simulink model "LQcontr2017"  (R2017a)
settings: Solver=VariableStepAuto  StartTime=0.0  StopTime=10.0  RelTol=1e-3
InitFcn:
  | initParams
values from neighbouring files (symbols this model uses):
  c = 8e-3    (= 0.008)    [initParams.m]
  g = 9.81    [initParams.m]
  L1 = 0.5    [initParams.m]
  m = 0.2    [initParams.m]
  R = 10    [initParams.m]
  ue = R*xe(3)    [initParams.m]
  x0 = [0.1;0;0.3]    [initParams.m]
  xe = [x1d;0;x1d*sqrt(g*m/c)]    [initParams.m]
undefined symbols (not defined in the file or in its folder): KLQ

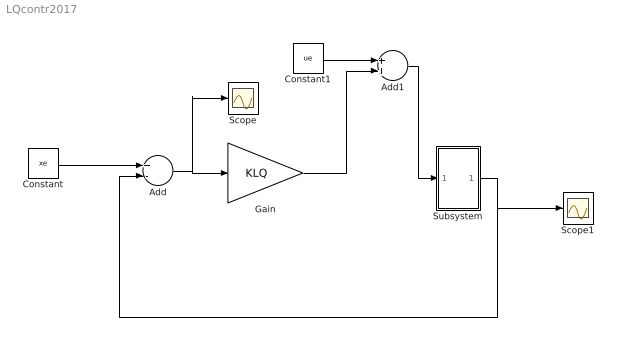
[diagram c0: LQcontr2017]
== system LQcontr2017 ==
  Add : Sum  Inputs=+-
  Add1 : Sum
  Constant : Constant  Value=xe
  Constant1 : Constant  Value=ue
  Gain : Gain  Gain=KLQ  Multiplication=Matrix(K*u) (u vector)
  Scope : Scope
  Scope1 : Scope
  Subsystem : Subsystem
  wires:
  Constant/1 -> Add/1
  Subsystem/1(x) -> Add/2, Scope1/1
  Add/1 -> Scope/1, Gain/1
  Constant1/1 -> Add1/1
  Gain/1 -> Add1/2
  Add1/1 -> Subsystem/1(u)

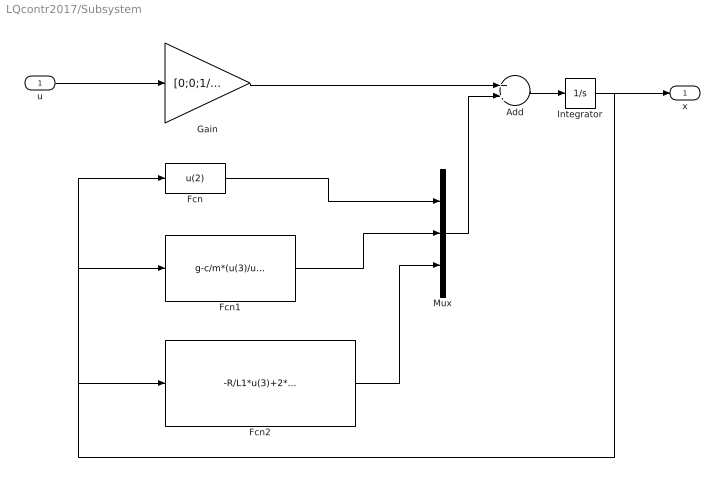
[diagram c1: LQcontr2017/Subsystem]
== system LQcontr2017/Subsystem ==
  u : Inport
  Add : Sum
  Fcn : Fcn  Expr=u(2)
  Fcn1 : Fcn  Expr=g-c/m*(u(3)/u(1))^2
  Fcn2 : Fcn  Expr=-R/L1*u(3)+2*c/L1*(u(2)*u(3)/(u(1))^2)
  Gain : Gain  Gain=[0;0;1/L1]  Multiplication=Matrix(K*u) (u vector)
  Integrator : Integrator  InitialCondition=x0
  Mux : Mux  Inputs=3
  x : Outport
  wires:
  Integrator/1 -> x/1, Fcn/1, Fcn1/1, Fcn2/1
  Gain/1 -> Add/1
  Fcn/1 -> Mux/1
  Fcn1/1 -> Mux/2
  Mux/1 -> Add/2
  Fcn2/1 -> Mux/3
  u/1 -> Gain/1
  Add/1 -> Integrator/1
